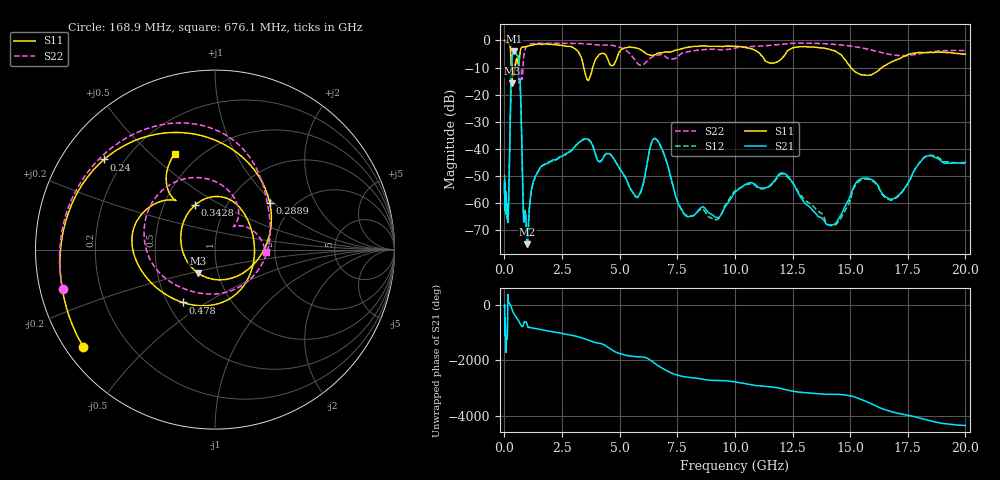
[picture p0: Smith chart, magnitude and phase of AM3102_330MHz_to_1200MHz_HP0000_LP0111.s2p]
! Date/Time: Tue, Sep 11, 2018 5:08 PM
! Network Analyzer: Agilent Technologies E8362B Rev: A.07.50.63
! Sweep from 0.010 to 20.000 GHz, 1601 Points, Sweep Type: LOG
! Power Supply: 4.950 V, 0.001 A
# Hz S DB R 50
!freq MagS11 AngS11 MagS21 AngS21 MagS12 AngS12 MagS22 AngS22
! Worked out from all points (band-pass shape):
!   1601 points, 10 MHz to 20 GHz, reference 50 ohm
!   highest |S21| = -3.99 dB at 420.4 MHz (marker M1); lowest = -75.2 dB at 998.1 MHz (marker M2)
!   |S21| within 3 dB of the highest: 323.4 MHz to 624.8 MHz (301.4 MHz wide, 63.6 % of centre)
!   lowest |S11| = -15.8 dB at 316.2 MHz (marker M3), VSWR 1.39, Z = 40 - j10.7 ohm
!   |S11| at or under -10 dB: 294.7 MHz to 463.8 MHz (169.1 MHz wide, 44.6 % of centre); 3.444 GHz to 3.83 GHz (386 MHz wide, 10.6 % of centre); 15.03 GHz to 16.38 GHz (1.35 GHz wide, 8.6 % of centre)
!   |S22| runs from -15.7 to -0.2 dB; largest |S21 - S12| = 0.011
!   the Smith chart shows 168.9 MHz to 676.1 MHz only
!   S11 on the Smith chart (normalised r, x): 168.9 MHz: 0.05, -0.33; 240 MHz: 0.13, +0.35; 288.9 MHz: 1.52, +0.95; 342.8 MHz: 0.72, +0.38; 478 MHz: 0.59, -0.40; 676.1 MHz: 0.37, +0.60
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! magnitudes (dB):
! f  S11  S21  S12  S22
! 10 MHz  0.0  -55.9  -49.4  -0.2
! 35.55 MHz  0.0  -61.5  -59.3  -0.4
! 126.4 MHz  -0.4  -62.3  -62.0  -0.9
! 168.9 MHz  -0.8  -64.3  -65.1  -1.2
! 240 MHz  -2.0  -35.7  -35.7  -1.8
! 288.9 MHz  -7.9  -14.7  -14.8  -3.8
! 316.2 MHz  -15.8  -7.9  -7.9  -7.1
! 342.8 MHz  -11.3  -5.6  -5.7  -10.0
! 420.4 MHz  -12.8  -4.0  -4.0  -10.6
! 447.2 MHz  -10.9  -4.1  -4.2  -9.1
! 478 MHz  -9.2  -4.4  -4.5  -7.9
! 676.1 MHz  -4.7  -13.7  -13.7  -11.0
! 829.3 MHz  -2.4  -64.9  -65.6  -7.0
! 998.1 MHz  -2.2  -75.2  -75.6  -1.9
! 1.59 GHz  -1.4  -46.5  -46.6  -1.0
! 3.582 GHz  -14.2  -36.3  -36.3  -1.3
! 5.652 GHz  -2.6  -57.0  -57.2  -7.1
! 6.58 GHz  -5.0  -36.3  -36.4  -5.5
! 7.92 GHz  -2.6  -64.9  -64.6  -4.2
! 12.09 GHz  -6.1  -48.9  -49.3  -1.4
! 14.07 GHz  -3.2  -68.2  -67.9  -1.3
! 20 GHz  -5.1  -45.0  -45.4  -3.7
